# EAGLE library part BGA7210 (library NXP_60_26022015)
700 MHz to 3800 MHz high linearity variable gain amplifier
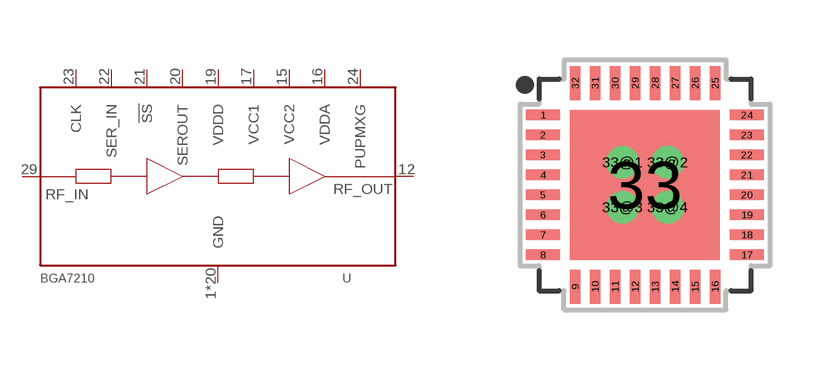
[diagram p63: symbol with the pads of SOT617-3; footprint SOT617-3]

Designator prefix U

## BGA7210  [SOT617-3]
1  GND  pwr
2  GND  pwr
3  GND  pwr
4  GND  pwr
5  GND  pwr
6  GND  pwr
7  GND  pwr
8  GND  pwr
9  GND  pwr
10  GND  pwr
12  RF_OUT  out
13  GND  pwr
14  GND  pwr
15  VCC2  pwr
16  VDDA  pwr
17  VCC1  pwr
18  GND  pwr
19  VDDD  pwr
20  SEROUT  out
21  !SS!  in
22  SER_IN  in
23  CLK  in
24  PUPMXG  in
25  GND  pwr
26  GND  pwr
27  GND  pwr
28  GND  pwr
29  RF_IN  in
31  GND  pwr
32  GND  pwr
33  GND  pwr

## Footprint SOT617-3 (pad centres in mm)
SOT617-3 HVQFN32: plastic thermal enhanced very thin quad flat package; no leads; 32 terminals; body 5 x 5 x 0.85 mm JEDEC: MO-220 IEC: -- JEITA: --
smd 0.85 x 0.27: 1 -2.55,1.75; 2 -2.55,1.25; 3 -2.55,0.75; 4 -2.55,0.25; 5 -2.55,-0.25; 6 -2.55,-0.75; 7 -2.55,-1.25; 8 -2.55,-1.75; 17 2.55,-1.75; 18 2.55,-1.25; 19 2.55,-0.75; 20 2.55,-0.25; 21 2.55,0.25; 22 2.55,0.75; 23 2.55,1.25; 24 2.55,1.75
smd 0.27 x 0.85: 9 -1.75,-2.55; 10 -1.25,-2.55; 11 -0.75,-2.55; 12 -0.25,-2.55; 13 0.25,-2.55; 14 0.75,-2.55; 15 1.25,-2.55; 16 1.75,-2.55; 25 1.75,2.55; 26 1.25,2.55; 27 0.75,2.55; 28 0.25,2.55; 29 -0.25,2.55; 30 -0.75,2.55; 31 -1.25,2.55; 32 -1.75,2.55
smd 3.75 x 3.75: 33 0,0
drill 0.3 pad 0.6: 33@1 -0.562,0.562; 33@2 0.562,0.562; 33@3 -0.562,-0.562; 33@4 0.562,-0.562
